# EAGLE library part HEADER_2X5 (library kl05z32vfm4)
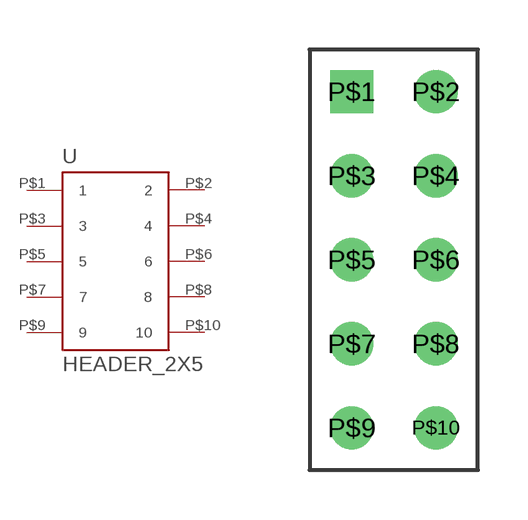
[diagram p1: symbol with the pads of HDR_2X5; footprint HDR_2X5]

Designator prefix -

## HEADER_2X5  [HDR_2X5]
P$1  1
P$2  2
P$3  3
P$4  4
P$5  5
P$6  6
P$7  7
P$8  8
P$9  9
P$10  10

## Footprint HDR_2X5 (pad centres in mm)
drill 0.8 square: P$1 -1.27,5.08
drill 0.8: P$2 1.27,5.08; P$3 -1.27,2.54; P$4 1.27,2.54; P$5 -1.27,0; P$6 1.27,0; P$7 -1.27,-2.54; P$8 1.27,-2.54; P$9 -1.27,-5.08; P$10 1.27,-5.08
